(* Logix 5000 AddOnInstructionDefinition export Banner_S15S_TH_PD_v4; software revision 33.03 *)

TYPE Banner_S15S_TH_Floating_Point :
STRUCT
   Temp_Value : REAL;
   Temp_Over_Threshold : SINT;
   Temp_Under_Threshold : SINT;
   Dew_Point_Value : REAL;
   Dew_Point_Over_Threshold : SINT;
   Dew_Point_Under_Threshold : SINT;
   Relative_Humidity_Value : REAL;
   Relative_Humidity_Over_Threshold : SINT;
   Relative_Humidity_Under_Threshold : SINT;
END_STRUCT
END_TYPE

TYPE Banner_S15S_TH_PDI_v4 :   // Process Data for a S15S-TH-KQ. This will include event information.
STRUCT
   Smart_Fahrenheit : Banner_S15S_TH_Smart_Sensor_v4;
   Smart_Celsius : Banner_S15S_TH_Smart_Sensor_v4;
   Floating_Fahrenheit : Banner_S15S_TH_Floating_Point;
   Floating_Celsius : Banner_S15S_TH_Floating_Point;
   DTI : SINT[16];
END_STRUCT
END_TYPE

TYPE Banner_S15S_TH_Smart_Sensor_v4 :
STRUCT
   Temp_Value : DINT;
   Temp_Scale : INT;
   Temp_Over_Threshold : SINT;
   Temp_Under_Threshold : SINT;
   Dew_Point_Value : DINT;
   Dew_Point_Scale : INT;
   Dew_Point_Over_Threshold : SINT;
   Dew_Point_Under_Threshold : SINT;
   Relative_Humidity_Value : DINT;
   Relative_Humidity_Scale : INT;
   Relative_Humidity_Over_Threshold : SINT;
   Relative_Humidity_Under_Threshold : SINT;
END_STRUCT
END_TYPE

ADD_ON_INSTRUCTION Banner_S15S_TH_Float_In_v4   (* revision 4.0 *)
// AOI the orientates the bytes for a floating point value.
VAR_IN_OUT
   Float : REAL; {required}
END_VAR
VAR_INPUT
   Sint0 : SINT; {required}
   Sint1 : SINT; {required}
   Sint2 : SINT; {required}
   Sint3 : SINT; {required}
END_VAR
VAR
   Temp_Byte : SINT[4]; {access None}
END_VAR

ROUTINE Logic   (* ladder *)
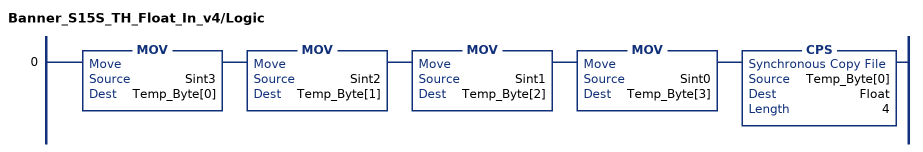
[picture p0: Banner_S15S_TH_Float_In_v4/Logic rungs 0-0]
   0: MOV(Sint3,Temp_Byte[0])MOV(Sint2,Temp_Byte[1])MOV(Sint1,Temp_Byte[2])MOV(Sint0,Temp_Byte[3])CPS(Temp_Byte[0],Float,4);
END_ROUTINE
END_ADD_ON_INSTRUCTION

ADD_ON_INSTRUCTION Banner_S15S_TH_PD_v4   (* revision 4.0, vendor Banner Engineering *)
// Take raw process data and convert it to usable values.
VAR_IN_OUT
   PD : Banner_S15S_TH_PDI_v4; {required}
   Operation_Mode : INT; {required}
END_VAR
VAR_INPUT
   Byte_Swap : BOOL; {required}
END_VAR
VAR
   Temp_Byte : SINT[16]; {access None}
   AOI_In_Status : Banner_S15S_TH_Float_In_v4[3]; {access None}
END_VAR

ROUTINE Logic   (* ladder *)
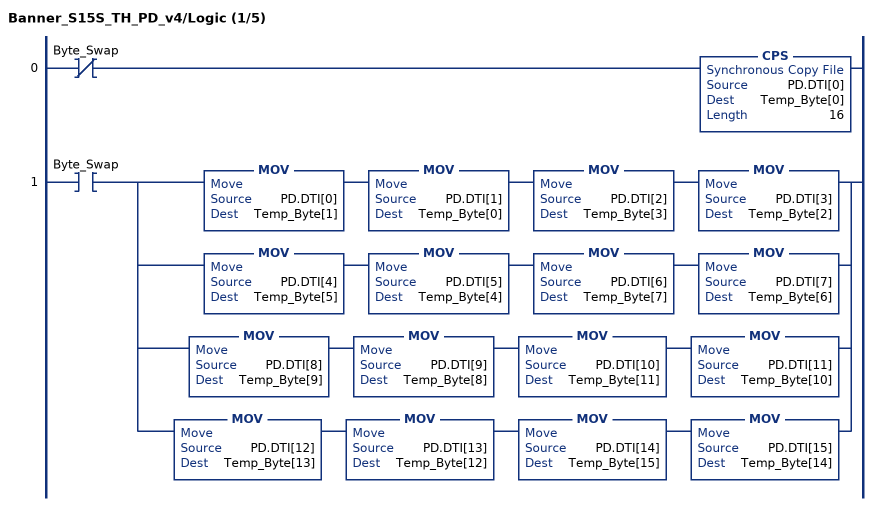
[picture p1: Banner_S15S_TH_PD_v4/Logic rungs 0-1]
   0: XIO(Byte_Swap)CPS(PD.DTI[0],Temp_Byte[0],16);
   1: XIC(Byte_Swap)[MOV(PD.DTI[0],Temp_Byte[1]) MOV(PD.DTI[1],Temp_Byte[0]) MOV(PD.DTI[2],Temp_Byte[3]) MOV(PD.DTI[3],Temp_Byte[2]) ,MOV(PD.DTI[4],Temp_Byte[5]) MOV(PD.DTI[5],Temp_Byte[4]) MOV(PD.DTI[6],Temp_Byte[7]) MOV(PD.DTI[7],Temp_Byte[6]) ,MOV(PD.DTI[8],Temp_Byte[9]) MOV(PD.DTI[9],Temp_Byte[8]) MOV(PD.DTI[10],Temp_Byte[11]) MOV(PD.DTI[11],Temp_Byte[10]) ,MOV(PD.DTI[12],Temp_Byte[13]) MOV(PD.DTI[13],Temp_Byte[12]) MOV(PD.DTI[14],Temp_Byte[15]) MOV(PD.DTI[15],Temp_Byte[14]) ];
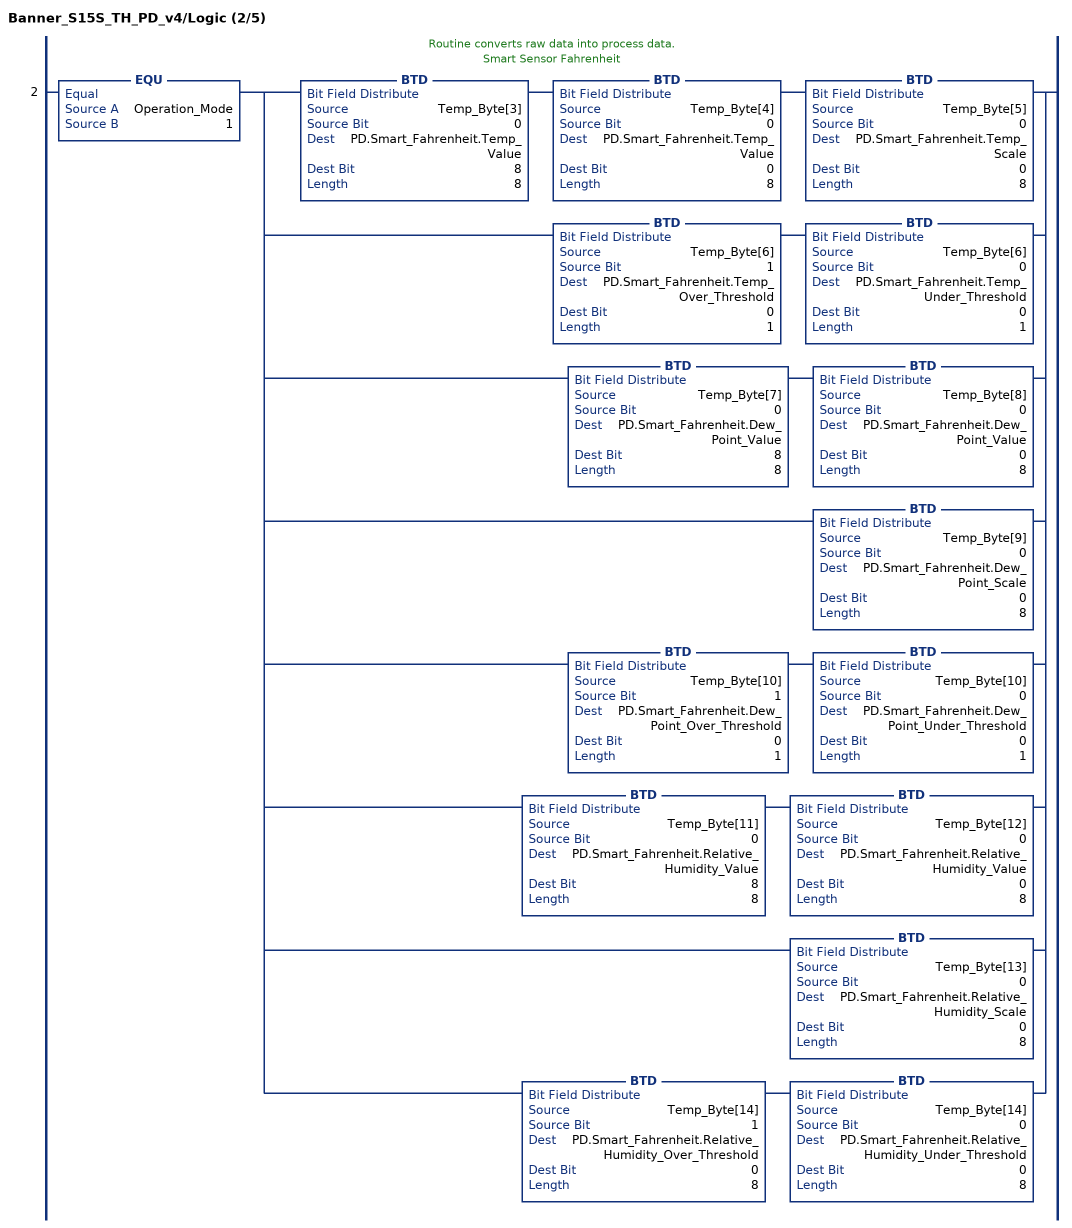
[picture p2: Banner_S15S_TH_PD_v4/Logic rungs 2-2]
   // Routine converts raw data into process data.
   // Smart Sensor Fahrenheit
   2: EQU(Operation_Mode,1)[BTD(Temp_Byte[3],0,PD.Smart_Fahrenheit.Temp_Value,8,8) BTD(Temp_Byte[4],0,PD.Smart_Fahrenheit.Temp_Value,0,8) BTD(Temp_Byte[5],0,PD.Smart_Fahrenheit.Temp_Scale,0,8) ,BTD(Temp_Byte[6],1,PD.Smart_Fahrenheit.Temp_Over_Threshold,0,1) BTD(Temp_Byte[6],0,PD.Smart_Fahrenheit.Temp_Under_Threshold,0,1) ,BTD(Temp_Byte[7],0,PD.Smart_Fahrenheit.Dew_Point_Value,8,8) BTD(Temp_Byte[8],0,PD.Smart_Fahrenheit.Dew_Point_Value,0,8) ,BTD(Temp_Byte[9],0,PD.Smart_Fahrenheit.Dew_Point_Scale,0,8) ,BTD(Temp_Byte[10],1,PD.Smart_Fahrenheit.Dew_Point_Over_Threshold,0,1) BTD(Temp_Byte[10],0,PD.Smart_Fahrenheit.Dew_Point_Under_Threshold,0,1) ,BTD(Temp_Byte[11],0,PD.Smart_Fahrenheit.Relative_Humidity_Value,8,8) BTD(Temp_Byte[12],0,PD.Smart_Fahrenheit.Relative_Humidity_Value,0,8) ,BTD(Temp_Byte[13],0,PD.Smart_Fahrenheit.Relative_Humidity_Scale,0,8) ,BTD(Temp_Byte[14],1,PD.Smart_Fahrenheit.Relative_Humidity_Over_Threshold,0,8) BTD(Temp_Byte[14],0,PD.Smart_Fahrenheit.Relative_Humidity_Under_Threshold,0,8) ];
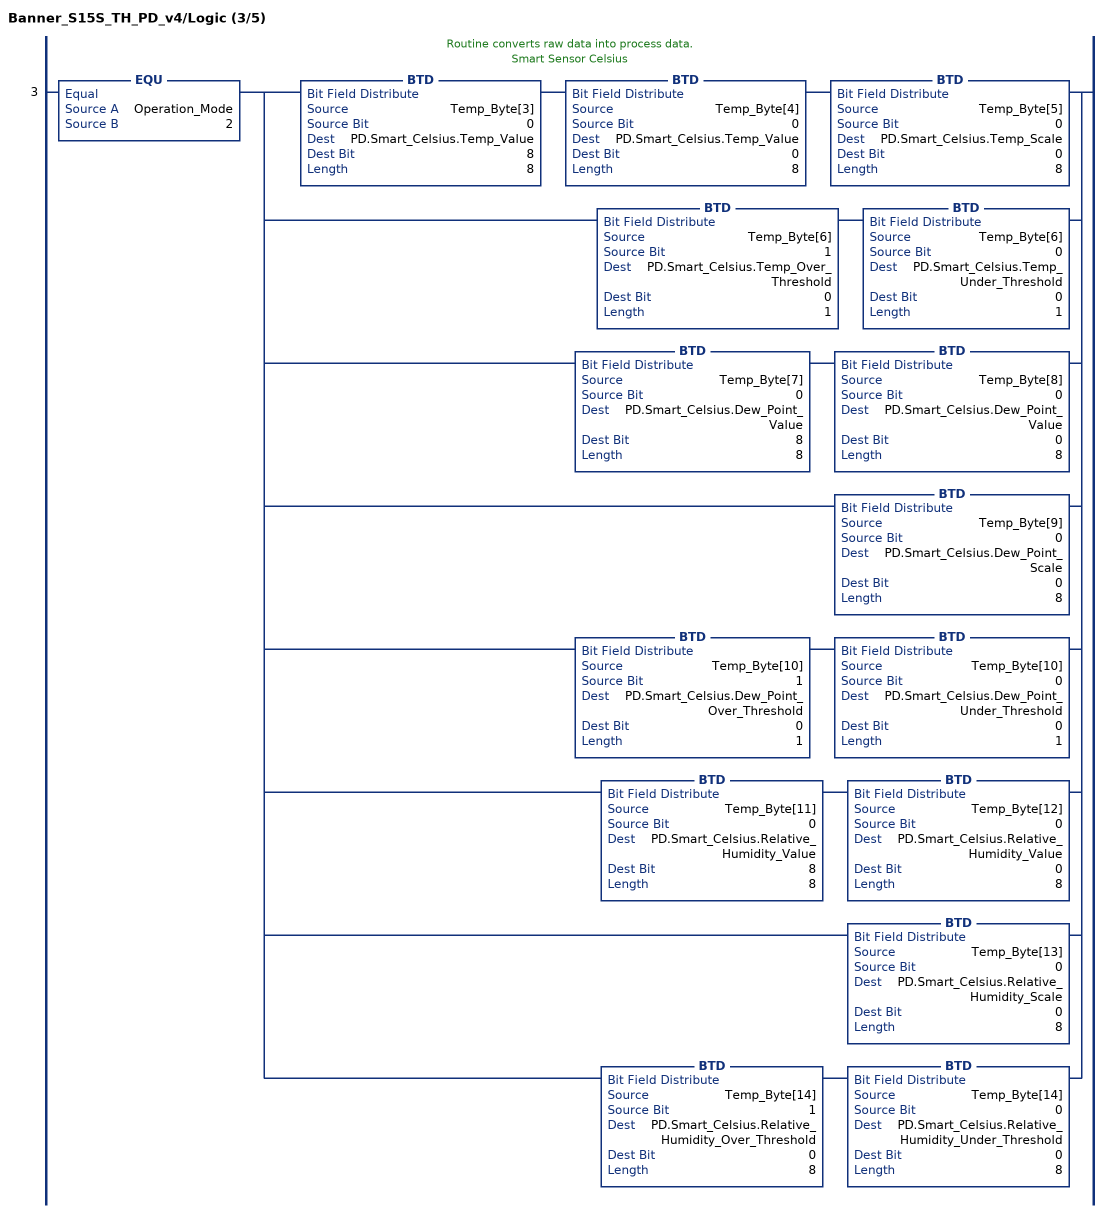
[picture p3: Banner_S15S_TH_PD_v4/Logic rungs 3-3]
   // Routine converts raw data into process data.
   // Smart Sensor Celsius
   3: EQU(Operation_Mode,2)[BTD(Temp_Byte[3],0,PD.Smart_Celsius.Temp_Value,8,8) BTD(Temp_Byte[4],0,PD.Smart_Celsius.Temp_Value,0,8) BTD(Temp_Byte[5],0,PD.Smart_Celsius.Temp_Scale,0,8) ,BTD(Temp_Byte[6],1,PD.Smart_Celsius.Temp_Over_Threshold,0,1) BTD(Temp_Byte[6],0,PD.Smart_Celsius.Temp_Under_Threshold,0,1) ,BTD(Temp_Byte[7],0,PD.Smart_Celsius.Dew_Point_Value,8,8) BTD(Temp_Byte[8],0,PD.Smart_Celsius.Dew_Point_Value,0,8) ,BTD(Temp_Byte[9],0,PD.Smart_Celsius.Dew_Point_Scale,0,8) ,BTD(Temp_Byte[10],1,PD.Smart_Celsius.Dew_Point_Over_Threshold,0,1) BTD(Temp_Byte[10],0,PD.Smart_Celsius.Dew_Point_Under_Threshold,0,1) ,BTD(Temp_Byte[11],0,PD.Smart_Celsius.Relative_Humidity_Value,8,8) BTD(Temp_Byte[12],0,PD.Smart_Celsius.Relative_Humidity_Value,0,8) ,BTD(Temp_Byte[13],0,PD.Smart_Celsius.Relative_Humidity_Scale,0,8) ,BTD(Temp_Byte[14],1,PD.Smart_Celsius.Relative_Humidity_Over_Threshold,0,8) BTD(Temp_Byte[14],0,PD.Smart_Celsius.Relative_Humidity_Under_Threshold,0,8) ];
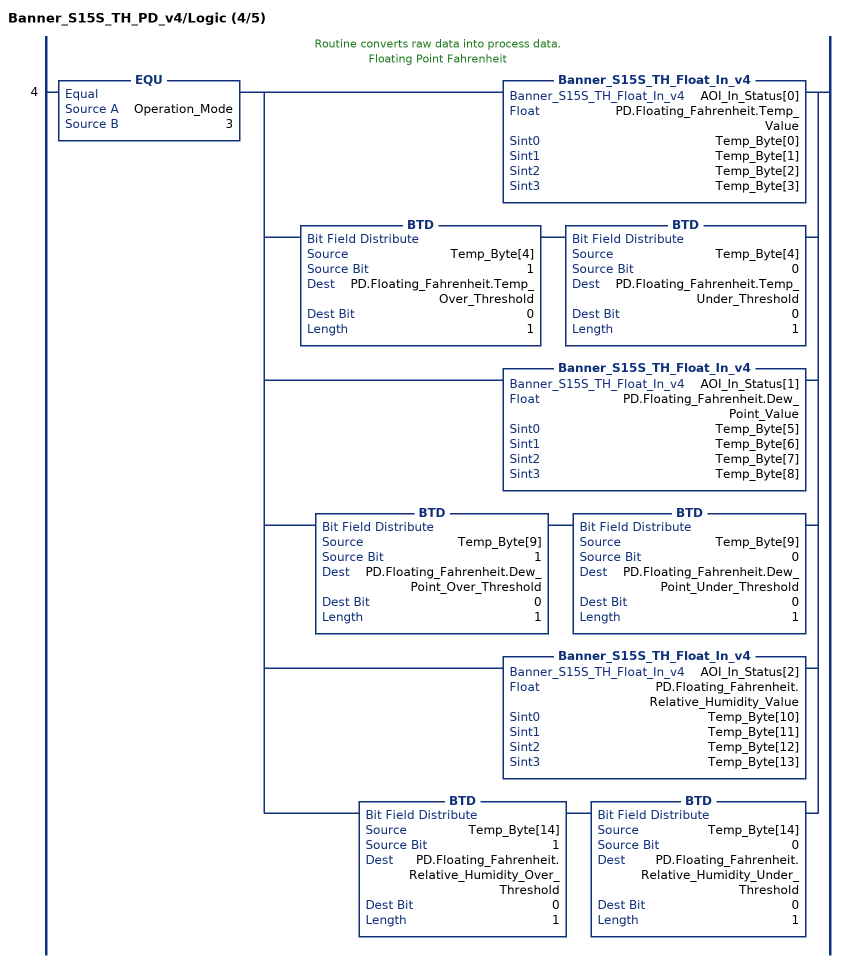
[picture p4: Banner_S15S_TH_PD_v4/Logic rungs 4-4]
   // Routine converts raw data into process data.
   // Floating Point Fahrenheit
   4: EQU(Operation_Mode,3)[Banner_S15S_TH_Float_In_v4(AOI_In_Status[0],PD.Floating_Fahrenheit.Temp_Value,Temp_Byte[0],Temp_Byte[1],Temp_Byte[2],Temp_Byte[3]) ,BTD(Temp_Byte[4],1,PD.Floating_Fahrenheit.Temp_Over_Threshold,0,1) BTD(Temp_Byte[4],0,PD.Floating_Fahrenheit.Temp_Under_Threshold,0,1) ,Banner_S15S_TH_Float_In_v4(AOI_In_Status[1],PD.Floating_Fahrenheit.Dew_Point_Value,Temp_Byte[5],Temp_Byte[6],Temp_Byte[7],Temp_Byte[8]) ,BTD(Temp_Byte[9],1,PD.Floating_Fahrenheit.Dew_Point_Over_Threshold,0,1) BTD(Temp_Byte[9],0,PD.Floating_Fahrenheit.Dew_Point_Under_Threshold,0,1) ,Banner_S15S_TH_Float_In_v4(AOI_In_Status[2],PD.Floating_Fahrenheit.Relative_Humidity_Value,Temp_Byte[10],Temp_Byte[11],Temp_Byte[12],Temp_Byte[13]) ,BTD(Temp_Byte[14],1,PD.Floating_Fahrenheit.Relative_Humidity_Over_Threshold,0,1) BTD(Temp_Byte[14],0,PD.Floating_Fahrenheit.Relative_Humidity_Under_Threshold,0,1) ];
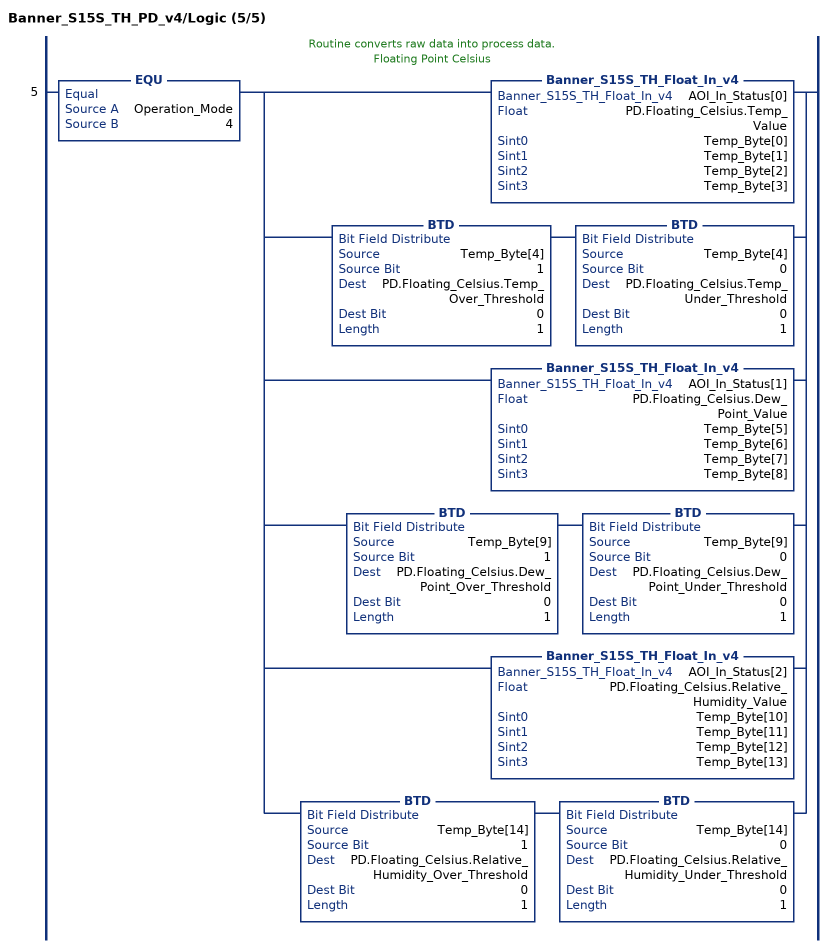
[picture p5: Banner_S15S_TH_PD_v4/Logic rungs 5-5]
   // Routine converts raw data into process data.
   // Floating Point Celsius
   5: EQU(Operation_Mode,4)[Banner_S15S_TH_Float_In_v4(AOI_In_Status[0],PD.Floating_Celsius.Temp_Value,Temp_Byte[0],Temp_Byte[1],Temp_Byte[2],Temp_Byte[3]) ,BTD(Temp_Byte[4],1,PD.Floating_Celsius.Temp_Over_Threshold,0,1) BTD(Temp_Byte[4],0,PD.Floating_Celsius.Temp_Under_Threshold,0,1) ,Banner_S15S_TH_Float_In_v4(AOI_In_Status[1],PD.Floating_Celsius.Dew_Point_Value,Temp_Byte[5],Temp_Byte[6],Temp_Byte[7],Temp_Byte[8]) ,BTD(Temp_Byte[9],1,PD.Floating_Celsius.Dew_Point_Over_Threshold,0,1) BTD(Temp_Byte[9],0,PD.Floating_Celsius.Dew_Point_Under_Threshold,0,1) ,Banner_S15S_TH_Float_In_v4(AOI_In_Status[2],PD.Floating_Celsius.Relative_Humidity_Value,Temp_Byte[10],Temp_Byte[11],Temp_Byte[12],Temp_Byte[13]) ,BTD(Temp_Byte[14],1,PD.Floating_Celsius.Relative_Humidity_Over_Threshold,0,1) BTD(Temp_Byte[14],0,PD.Floating_Celsius.Relative_Humidity_Under_Threshold,0,1) ];
END_ROUTINE
END_ADD_ON_INSTRUCTION
